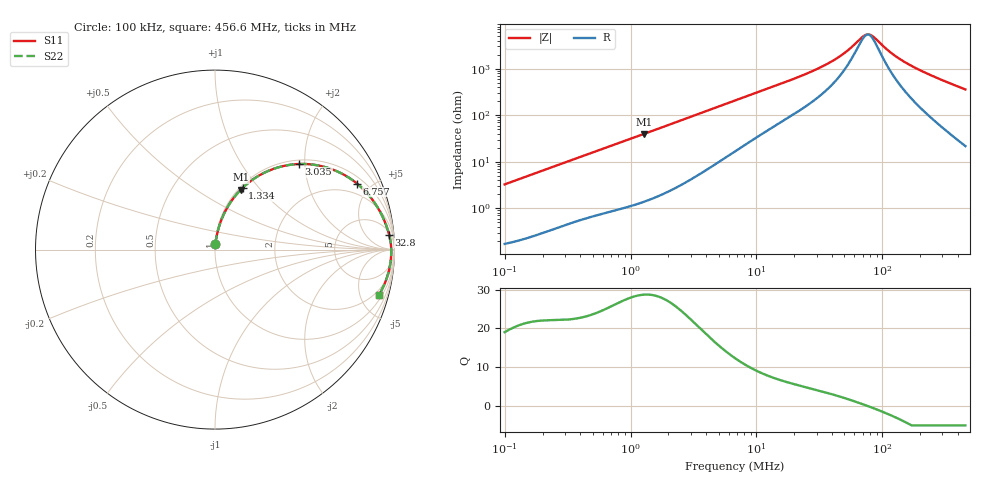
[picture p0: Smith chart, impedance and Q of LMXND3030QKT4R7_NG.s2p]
! LMXND3030QKT4R7_NG  S-PARAMETER MODEL  ( General Type )
! Model Generated by TAIYO YUDEN Corporation (http://www.ty-top.com)
! Version 1.0
! TAIYO YUDEN Control No. 191023NI43SB-FBB
! Copyright(c) 2019 TAIYO YUDEN CO.,LTD. All Rights Reserved.
! Product Description (link to TY-COMPAS)
! https://ds.yuden.co.jp/TYCOMPAS/or/detail?pn=LMXND3030QKT4R7MNG&u=M
! Products Name : Inductors
! Characteristics :
!  Inductance : 4.7 uH , SRF(min) : 40 MHz , DC Resistance(max) : 0.144 Ohm
!  Rated Current : Saturation :1020 mA , Temp Rise : 1040 mA
!  Case Size : 3.0 x 3.0 / 0.118 x 0.118 [mm/inch] , Thickness : 1.5 / 0.059 [mm/inch]
!  (Conditions: Temperature = 25 degC , DC Bias Current/Voltage = 0A / 0V)
! External Node Assignments :
!  1  o---GGG---o  2
! GND o---------o GND
! Frequency Range : 0.1MHz  -  456.598367MHz  [ 402 STEP ]
# MHz S RI R 50
! Freq[MHz].  S11 Real  S11 Imag  S21 Real  S21 Imag  S12 Real  S12 Imag  S22 Real  S22 Imag
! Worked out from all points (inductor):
!   401 points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, 100 kHz to 456.6 MHz, reference 50 ohm
!   read as one part in series: L = 5.17 uH near 104.3 kHz
!   highest Q = 28.7 at 1.279 MHz (marker M1), where L = 4.92 uH
!   self-resonance near 76.56 MHz
!   S11 on the Smith chart (normalised r, x): 100 kHz: 1.00, +0.07; 1.334 MHz: 1.03, +0.82; 3.035 MHz: 1.08, +1.86; 6.757 MHz: 1.33, +4.11; 32.8 MHz: 7, +21; 456.6 MHz: 1.43, -7.15
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0.1  0.00276 0.0324  0.9972 -0.0324  0.9972 -0.0324  0.00276 0.0324
0.410178  0.0219 0.1262  0.9781 -0.1262  0.9781 -0.1262  0.0219 0.1262
0.788108  0.0644 0.2273  0.9356 -0.2273  0.9356 -0.2273  0.0644 0.2273
1.279408  0.1439 0.334  0.8561 -0.334  0.8561 -0.334  0.1439 0.334
1.334464  0.154 0.3439  0.846 -0.3439  0.846 -0.3439  0.154 0.3439
1.682457  0.2205 0.3972  0.7795 -0.3972  0.7795 -0.3972  0.2205 0.3972
3.03467  0.4671 0.4769  0.5329 -0.4769  0.5329 -0.4769  0.4671 0.4769
4.341518  0.6323 0.4543  0.3677 -0.4543  0.3677 -0.4543  0.6323 0.4543
6.757206  0.7914 0.3678  0.2086 -0.3678  0.2086 -0.3678  0.7914 0.3678
6.901063  0.7973 0.3629  0.2027 -0.3629  0.2027 -0.3629  0.7973 0.3629
12.44754  0.9084 0.2311  0.0916 -0.2311  0.0916 -0.2311  0.9084 0.2311
27.71655  0.9644 0.104  0.0356 -0.104  0.0356 -0.104  0.9644 0.104
32.80423  0.97 0.0839  0.03 -0.0839  0.03 -0.0839  0.97 0.0839
47.93016  0.9781 0.0439  0.0219 -0.0439  0.0219 -0.0439  0.9781 0.0439
68.57079  0.9815 0.0101  0.0185 -0.0101  0.0185 -0.0101  0.9815 0.0101
74.59925  0.9819 0.00238  0.0181 -0.00238  0.0181 -0.00238  0.9819 0.00238
79.46593  0.982 -0.00344  0.018 0.00344  0.018 0.00344  0.982 -0.00344
84.6501  0.9821 -0.00928  0.0179 0.00928  0.0179 0.00928  0.9821 -0.00928
113.6871  0.9813 -0.0375  0.0187 0.0375  0.0187 0.0375  0.9813 -0.0375
143.3337  0.9791 -0.0618  0.0209 0.0618  0.0209 0.0618  0.9791 -0.0618
196.5988  0.9729 -0.1001  0.0271 0.1001  0.0271 0.1001  0.9729 -0.1001
456.5984  0.9147 -0.2507  0.0853 0.2507  0.0853 0.2507  0.9147 -0.2507
